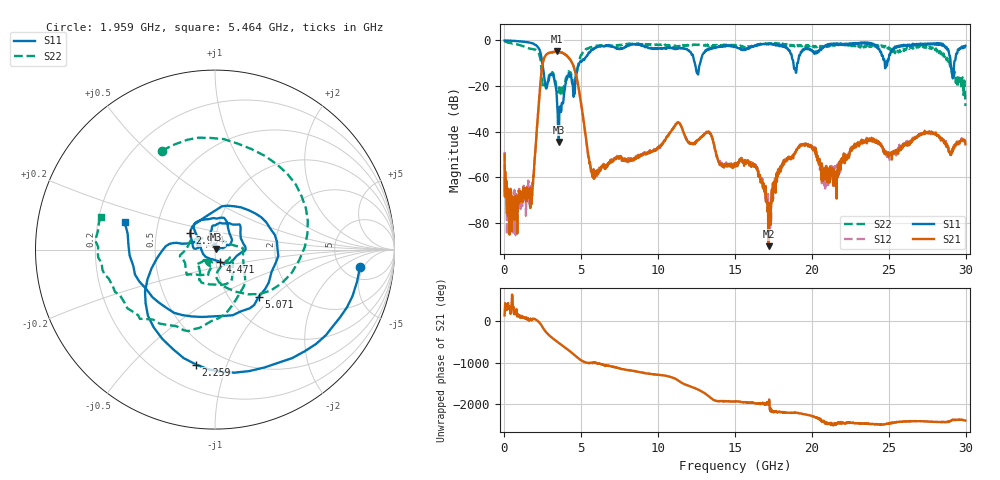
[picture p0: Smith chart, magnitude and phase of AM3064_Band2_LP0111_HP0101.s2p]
# Hz S DB R 50.0
!freq dBS11 angS11 dBS21 angS21 dBS12 angS12 dBS22 angS22
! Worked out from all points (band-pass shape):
!   1600 points, 10 MHz to 29.98 GHz, reference 50 ohm
!   highest |S21| = -4.83 dB at 3.403 GHz (marker M1); lowest = -90.3 dB at 17.18 GHz (marker M2)
!   |S21| within 3 dB of the highest: 2.577 GHz to 4.197 GHz (1.62 GHz wide, 47.8 % of centre)
!   lowest |S11| = -44.6 dB at 3.534 GHz (marker M3), VSWR 1.01, Z = 50.5 + j0.249 ohm
!   |S11| at or under -10 dB: 2.453 GHz to 4.869 GHz (2.416 GHz wide, 66 % of centre); 12.38 GHz to 12.73 GHz (343 MHz wide, 2.73 % of centre); 18.8 GHz to 19.05 GHz (249.8 MHz wide, 1.32 % of centre)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
!   |S22| runs from -28.8 to -0.2 dB; largest |S21 - S12| = 0.018
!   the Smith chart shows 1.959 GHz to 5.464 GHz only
!   S11 on the Smith chart (normalised r, x): 1.959 GHz: 7.29, -4.20; 2.259 GHz: 0.35, -0.78; 2.934 GHz: 0.75, +0.14; 4.471 GHz: 1.05, -0.14; 5.071 GHz: 1.36, -0.82; 5.464 GHz: 0.32, +0.13
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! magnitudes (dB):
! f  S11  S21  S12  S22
! 10 MHz  0.0  -50.0  -48.9  -0.2
! 572.3 MHz  -0.2  -76.8  -84.4  -1.4
! 1.959 GHz  -1.8  -52.8  -52.8  -4.1
! 2.259 GHz  -3.8  -25.6  -25.5  -6.0
! 2.934 GHz  -15.6  -5.5  -5.4  -14.5
! 3.403 GHz  -24.8  -4.8  -5.0  -21.6
! 3.534 GHz  -44.6  -5.1  -5.0  -22.0
! 4.471 GHz  -22.7  -11.0  -10.8  -20.4
! 5.015 GHz  -9.4  -29.1  -29.0  -6.4
! 5.071 GHz  -8.9  -31.8  -31.7  -5.7
! 5.464 GHz  -5.6  -50.8  -51.0  -3.6
! 10 GHz  -3.6  -47.3  -47.0  -2.0
! 11.31 GHz  -3.2  -36.2  -36.1  -2.7
! 15 GHz  -2.6  -55.1  -54.3  -2.0
! 16.34 GHz  -2.3  -55.3  -55.2  -2.4
! 17.18 GHz  -1.7  -90.3  -75.4  -1.7
! 18.17 GHz  -2.4  -52.5  -54.0  -2.1
! 19.99 GHz  -4.2  -46.7  -47.1  -2.2
! 20.95 GHz  -2.4  -61.0  -59.7  -2.3
! 25 GHz  -8.1  -51.1  -49.7  -3.1
! 28.31 GHz  -1.7  -42.4  -42.1  -4.7
! 29.98 GHz  -2.3  -45.6  -44.5  -28.8
